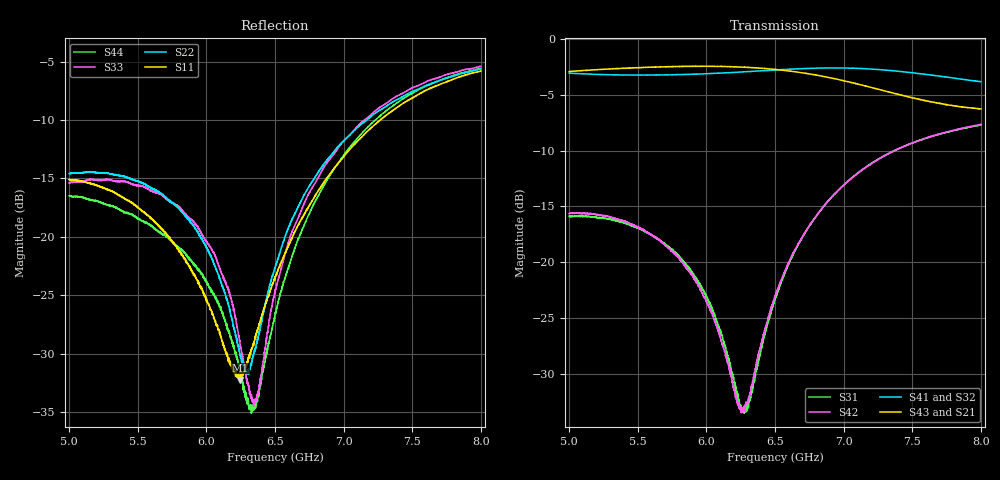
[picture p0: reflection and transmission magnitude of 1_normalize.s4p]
!Keysight Technologies,N5225A,MY51451420,A.10.40.12
!Date: Wednesday, May 11, 2016 10:29:44
!Correction: S11(Full 4 Port(1,2,3,4))
!S12(Full 4 Port(1,2,3,4))
!S13(Full 4 Port(1,2,3,4))
!S14(Full 4 Port(1,2,3,4))
!S21(Full 4 Port(1,2,3,4))
!S22(Full 4 Port(1,2,3,4))
!S23(Full 4 Port(1,2,3,4))
!S24(Full 4 Port(1,2,3,4))
!S31(Full 4 Port(1,2,3,4))
!S32(Full 4 Port(1,2,3,4))
!S33(Full 4 Port(1,2,3,4))
!S34(Full 4 Port(1,2,3,4))
!S41(Full 4 Port(1,2,3,4))
!S42(Full 4 Port(1,2,3,4))
!S43(Full 4 Port(1,2,3,4))
!S44(Full 4 Port(1,2,3,4))
!S4P File: Measurements: <S11,S12,S13,S14>,
!<S21,S22,S23,S24>,
!<S31,S32,S33,S34>,
!<S41,S42,S43,S44>:
# Hz S  dB  R 50
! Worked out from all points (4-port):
!   3201 points, 5 GHz to 8 GHz, reference 50 ohm
!   strongest paths, dB at 5 GHz, 5.75 GHz, 6.5 GHz, 7.25 GHz, 8 GHz:
!     S43: -2.9, -2.5, -2.8, -4.5, -6.3
!     S21: -3.0, -2.5, -2.8, -4.5, -6.1
!     S41: -3.1, -3.2, -2.8, -2.8, -3.8
!     S32: -3.1, -3.3, -2.8, -2.9, -3.9
!     S42: -15.6, -19.0, -23.0, -10.8, -7.7
!     S31: -15.9, -18.9, -23.3, -10.8, -7.7
!   lowest |S11| = -32.3 dB at 6.247 GHz (marker M1), VSWR 1.05, Z = 52.2 + j1.09 ohm
!   |S11| at or under -10 dB: start of sweep to 7.268 GHz
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5e9  -15.11 -169.9  -3.02 -80.2  -15.88 -17.1  -3.08 -175.1
     -3.01 -80.3  -14.60 65.2  -3.10 -56.8  -15.64 100.9
     -15.87 -17.1  -3.10 -56.8  -15.40 41.9  -2.93 31.2
     -3.08 -175.1  -15.63 100.9  -2.94 31.2  -16.50 43.8
5.816562e9  -21.57 133.5  -2.51 -107.9  -19.66 -29.1  -3.21 157.5
            -2.51 -108.0  -17.82 42.7  -3.27 -64.0  -19.90 105.6
            -19.67 -29.3  -3.27 -64.0  -17.57 37.4  -2.48 21.5
            -3.21 157.5  -19.91 105.5  -2.49 21.6  -21.12 41.2
6.246875e9  -32.26 25.3  -2.57 -123.6  -32.97 13.2  -2.98 141.9
            -2.57 -123.7  -30.15 -13.4  -2.97 -69.5  -32.95 167.2
            -32.93 12.6  -2.97 -69.5  -29.42 59.6  -2.53 15.6
            -2.98 141.9  -32.90 167.4  -2.53 15.6  -31.80 74.0
6.359375e9  -28.48 -27.1  -2.65 -127.8  -29.88 74.7  -2.90 137.5
            -2.65 -127.8  -29.43 -86.2  -2.89 -71.3  -29.38 -133.5
            -29.83 74.3  -2.88 -71.4  -33.88 135.3  -2.60 13.9
            -2.91 137.5  -29.45 -133.6  -2.61 14.0  -34.44 138.2
6.591875e9  -20.91 -73.7  -2.93 -136.3  -20.37 94.0  -2.74 127.9
            -2.94 -136.4  -19.41 -131.0  -2.75 -75.7  -20.18 -111.7
            -20.38 94.0  -2.75 -75.6  -20.67 -165.1  -2.87 10.4
            -2.74 127.9  -20.19 -111.5  -2.87 10.5  -22.83 -163.8
6.876875e9  -14.96 -105.9  -3.49 -146.1  -14.67 86.8  -2.62 115.2
            -3.49 -146.2  -13.48 -145.4  -2.69 -81.7  -14.63 -111.8
            -14.67 86.9  -2.69 -81.7  -13.71 -159.9  -3.43 6.7
            -2.62 115.2  -14.65 -111.6  -3.44 6.7  -15.17 -158.2
8e9  -5.82 176.1  -6.12 -168.6  -7.72 47.2  -3.85 65.8
     -6.11 -168.6  -5.61 -164.6  -3.93 -103.4  -7.68 -124.3
     -7.72 47.3  -3.93 -103.3  -5.40 -169.9  -6.28 11.0
     -3.85 65.7  -7.67 -124.3  -6.28 11.0  -5.59 -172.2
